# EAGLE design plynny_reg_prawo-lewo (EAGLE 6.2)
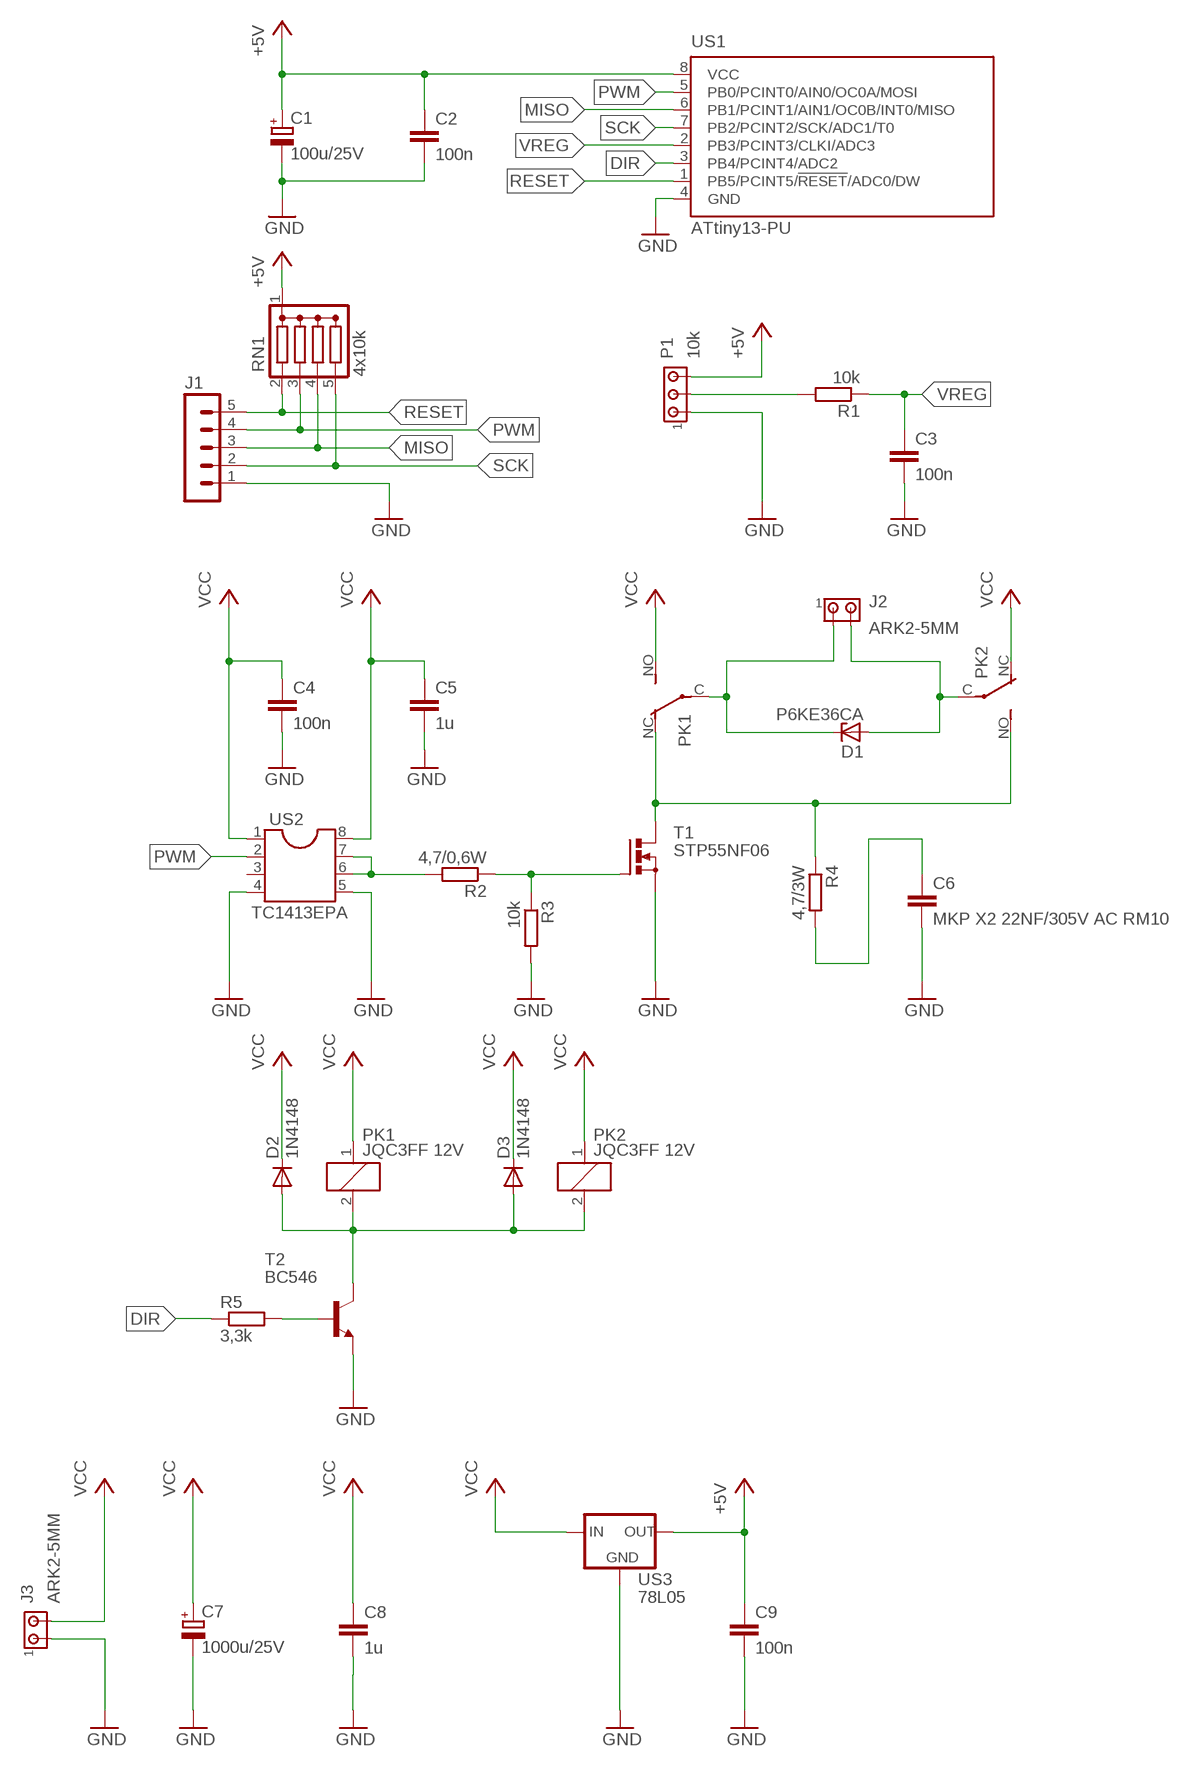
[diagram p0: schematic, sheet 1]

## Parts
C1  100u/25V  CPOL-EUE2.5-6  [E2,5-6]
C2  100n  C-EU050-025X075  [C050-025X075]
C3  100n  C-EU050-025X075  [C050-025X075]
C4  100n  C-EU050-025X075  [C050-025X075]
C5  1u  C-EU050-055X075  [C050-055X075]
C6  MKP X2 22NF/305V AC RM10  C-EU102-054X133  [C102-054X133]
C7  1000u/25V  CPOL-EUE5-10.5  [E5-10,5]
C8  1u  C-EU050-055X075  [C050-055X075]
C9  100n  C-EU050-025X075  [C050-025X075]
D1  P6KE36CA  ZENER-DIODEC1702-15  [C1702-15]
D2  1N4148  1N4148DO35-10  [DO35-10]
D3  1N4148  1N4148DO35-10  [DO35-10]
J1  MA05-1  [MA05-1]
J2  ARK2-5MM  [2PIN-5MM]
J3  ARK2-5MM  [2PIN-5MM]
P1  10k  ARK3-5MM  [3PIN-5MM]
PK1  JQC3FF 12V  PK_POJED-JQC-3FG  [PK_POJED_JQC-3FG]
PK2  JQC3FF 12V  PK_POJED-JQC-3FG  [PK_POJED_JQC-3FG]
R1  10k  R-EU_0207/7  [0207/7]
R2  4,7/0,6W  R-EU_0207/12  [0207/12]
R3  10k  R-EU_0207/7  [0207/7]
R4  4,7/3W  R-EU_R_18MM  [R_18MM]
R5  3,3k  R-EU_0207/7  [0207/7]
RN1  4x10k  DRAB_REZ_1X4  [RN-5]
T1  STP55NF06  BUZ11BV  [TO220BV]
T2  BC546  BC546A  [TO92-EBC]
US1  ATtiny13-PU  TINY13-20PU  [DIL08]
US2  TC1413EPA  DIL8  [DIL08]
US3  78L05  78LXX  [78LXX]

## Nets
+5V: C1.+ C2.1 C9.1 P1.P$3 RN1.1(C) US1.8(VCC) US3.OUT
DIR: R5.1 US1.3(PB4/PCINT4/ADC2)
GND: C1.- C2.2 C3.2 C4.2 C5.2 C6.2 C7.- C8.2 C9.2 J1.1 J3.P$1 P1.P$1 R3.2 T1.S T2.E US1.4(GND) US2.4 US2.5 US3.GND
MISO: J1.3 RN1.4 US1.6(PB1/PCINT1/AIN1/OC0B/INT0/MISO)
N$1: P1.P$2 R1.2
N$2: R2.2 US2.6 US2.7
N$3: PK1.NC PK2.NO R4.P$1 T1.D
N$4: C6.1 R4.P$2
N$5: R2.1 R3.1 T1.G
N$6: D1.C J2.P$1 PK1.C(COM)
N$7: D1.A J2.P$2 PK2.C(COM)
N$8: R5.2 T2.B
N$9: D2.A D3.A PK1.2 PK2.2 T2.C
PWM: J1.4 RN1.3 US1.5(PB0/PCINT0/AIN0/OC0A/MOSI) US2.2
RESET: J1.5 RN1.2 US1.1(PB5/PCINT5/!RESET!/ADC0/DW)
SCK: J1.2 RN1.5 US1.7(PB2/PCINT2/SCK/ADC1/T0)
VCC: C4.1 C5.1 C7.+ C8.1 D2.C D3.C J3.P$2 PK1.1 PK1.NO PK2.1 PK2.NC US2.1 US2.8 US3.IN
VREG: C3.1 R1.1 US1.2(PB3/PCINT3/CLKI/ADC3)
Unconnected: US2.3

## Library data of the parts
C1 C7 = rcl:CPOL-EU: POLARIZED CAPACITOR, European symbol
C2-C6 C8 C9 = rcl:C-EU: CAPACITOR, European symbol
D1 = diode:ZENER-DIODE: Z-Diode
D2 D3 = diode:1N4148: DIODE
J1 = con-lstb:MA05-1: PIN HEADER; OC_FARNELL: unknown; OC_NEWARK: unknown
J2 J3 = zlacza_futrzak:ARK2: ARK 2
P1 = zlacza_futrzak:ARK3: ARK 3 Raster 5mm i 3,5mm
PK1 PK2 = inne_futrzak:PK_POJED
R1-R5 = rcl:R-EU_: RESISTOR, European symbol
RN1 = inne_futrzak:DRAB_REZ_1X4
T1 = transistor-power:BUZ11: N-CHANNEL MOS FET
T2 = transistor-npn:BC546*: NPN Transistor
US1 = atmel:TINY13: 8-bit AVR Microcontroller with 1K Bytes In-System Programmable Flash Source: http://www.atmel.com/dyn/resources/prod_documents/2535S.pdf; MPN: ATTINY13-20PU; OC_FARNELL: 9171550; OC_NEWARK: 96K6521
US2 = ic-package:DIL8: Dual In Line / Socket
US3 = v-reg:78LXX: VOLTAGE REGULATOR

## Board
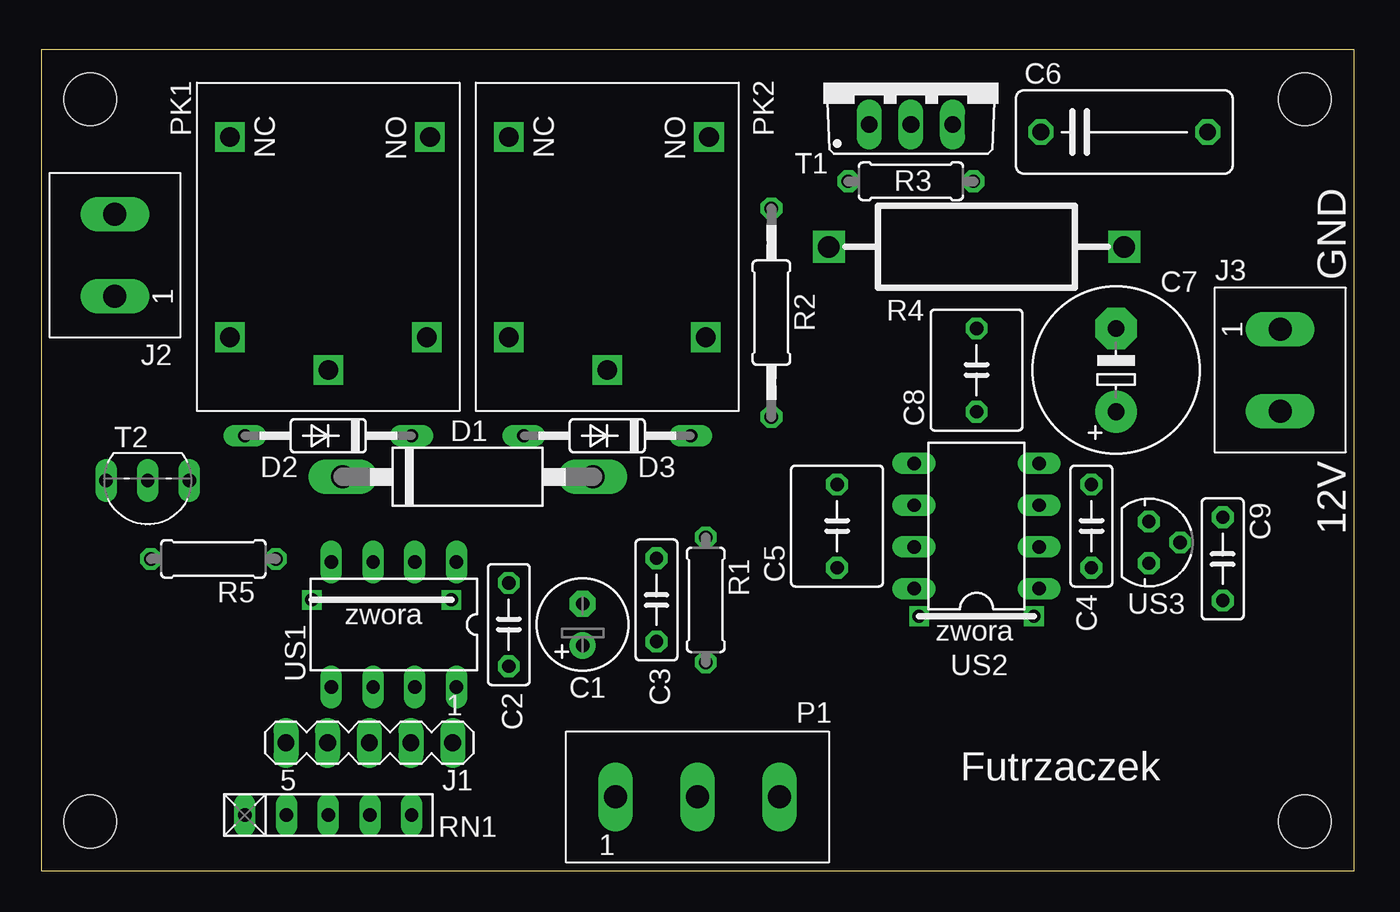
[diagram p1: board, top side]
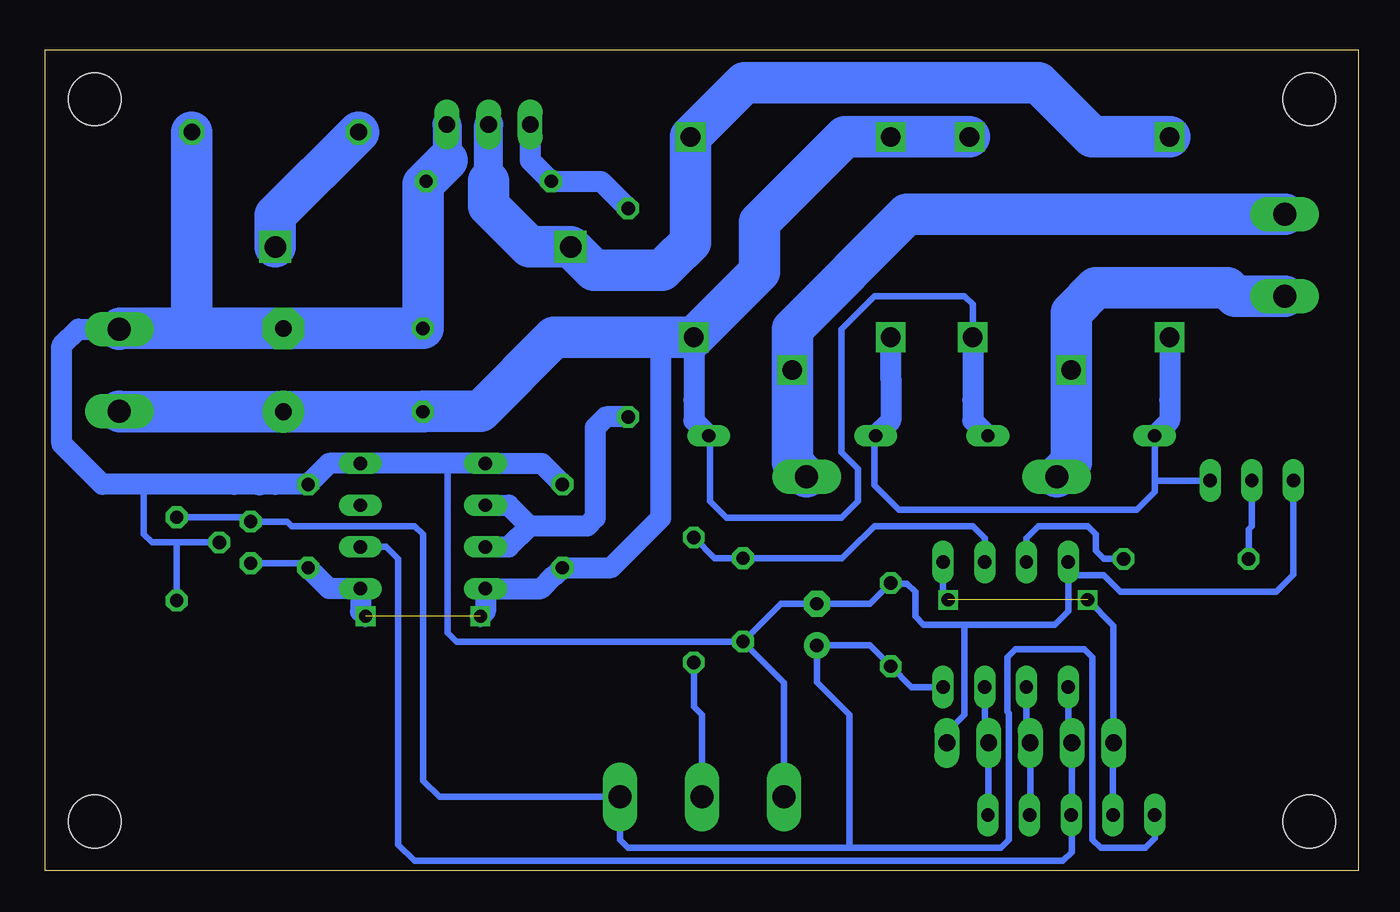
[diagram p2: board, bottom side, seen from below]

Size 80 x 50 mm. Coordinates in mm from the lower left corner, seen from the top.
Outline: 0,0 80,0 80,50 0,50 0,0
Copper layers (1*16): Top 0.035mm / dielectric 1.5mm / Bottom 0.035mm
Design rules: minimum track width 10mil, minimum drill 23mil, track to track 8mil, track to pad 8mil, pad to pad 8mil, via to via 8mil, smd to smd 8mil, copper to edge 10mil, drill to drill 8mil, minimum pad ring 10mil, minimum via ring 8mil, stop-mask expansion 4mil, vias tented up to drill 0mil, thermal gap 10mil
Holes 3.2 mm at 3,3 3,47 77,3 77,47

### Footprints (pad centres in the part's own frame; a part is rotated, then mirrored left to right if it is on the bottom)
E2,5-6 = drill 0.813 pad 1.6: + -1.27,0 | drill 0.813 pad 1.6 octagon: - 1.27,0
C050-025X075 = drill 0.813 octagon: 1 -2.54,0; 2 2.54,0
C050-055X075 = drill 0.813 octagon: 1 -2.54,0; 2 2.54,0
C102-054X133 = drill 1.016 octagon: 1 -5.08,0; 2 5.08,0
E5-10,5 = drill 1.016 pad 2.54: + -2.54,0 | drill 1.016 pad 2.54 octagon: - 2.54,0
C1702-15 = drill 1.397 long: A 7.62,0; C -7.62,0
DO35-10 = drill 0.813 long: A 5.08,0; C -5.08,0
MA05-1 = drill 1.016 long: 1 -5.08,0; 2 -2.54,0; 3 0,0; 4 2.54,0; 5 5.08,0
2PIN-5MM = drill 1.4 long: P$1 -2.5,0; P$2 2.5,0
3PIN-5MM = drill 1.4 long: P$1 -5,0; P$2 0,0; P$3 5,0
PK_POJED_JQC-3FG = drill 1.2 square: 1 5.5,6; 2 5.5,-6; C 7.5,0; NC -6.7,-6; NO -6.7,6.2
0207/7 = drill 0.813 octagon: 1 -3.81,0; 2 3.81,0
0207/12 = drill 0.813 octagon: 1 -6.35,0; 2 6.35,0
R_18MM = drill 1.3 square: P$1 -9,0; P$2 9,0
RN-5 = drill 0.813 long: 1 -5.08,0; 2 -2.54,0; 3 0,0; 4 2.54,0; 5 5.08,0
TO220BV = drill 1.016 long: D 0,-2.54; G -2.54,-2.54; S 2.54,-2.54
TO92-EBC = drill 0.813 long: B 0,-1.27; C -2.54,-1.27; E 2.54,-1.27
DIL08 = drill 0.813 long: 1 -3.81,-3.81; 2 -1.27,-3.81; 3 1.27,-3.81; 4 3.81,-3.81; 5 3.81,3.81; 6 1.27,3.81; 7 -1.27,3.81; 8 -3.81,3.81
78LXX = drill 0.813 octagon: GND 0,1.905; IN 1.27,0; OUT -1.27,0

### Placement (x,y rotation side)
C1  33,15 90 top
C2  28.5,15 90 top
C3  37.5,16.5 270 top
C4  64,21 90 top
C5  48.5,21 90 top
C6  66,45 0 top
C7  65.5,30.5 90 top
C8  57,30.5 90 top
C9  72,19 270 top
D1  26,24 0 top
D2  17.5,26.5 180 top
D3  34.5,26.5 180 top
J1  20,7.8 180 top
J2  4.5,37.5 90 top
J3  75.5,30.5 270 top
P1  40,4.5 0 top
PK1  17.5,38 270 top
PK2  34.5,38 270 top
R1  40.5,16.5 270 top
R2  44.5,34 270 top
R3  53,42 0 top
R4  57,38 0 top
R5  10.5,19 180 top
RN1  17.5,3.4 0 top
T1  53,48 0 top
T2  6.5,22.5 180 top
US1  21.5,15 180 top
US2  57,21 90 top
US3  67.5,20 270 top

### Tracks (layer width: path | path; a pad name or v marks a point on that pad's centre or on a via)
+5V
  Bottom 0.406: US1.8 27.23,11.19 C2.1 29.77,13.73 C1.+ 33,11.5 31,9.5 31,1.4 | RN1.1 12.42,1.98 13,1.4 15.7,1.4 16.2,1.9 16.2,13 16.7,13.5 20.3,13.5 20.9,13.5 21.4,13 21.4,9.7 21.3,9.6 21.3,1.9 21.8,1.4 31,1.4 | 31,1.4 44.5,1.4 45,1.9 P1.P$3 56,4.5 57,5.5 57,20.5 57.5,21 65,21 65.27,21.27 US3.OUT 67.77,21.54 C9.1
DIR
  Bottom 0.406: US1.3 20.23,20.27 19.5,21 16.5,21 16,20.5 16,19.5 15.5,19 R5.1
GND
  Bottom 0.406: US1.4 17.69,18 | 17.69,18 17.69,17.31 17.69,15.81 18.5,15 24,15 | 24,15 26.5,15 27,15.5 27,17 27.5,17.5 28.46,17.5 C2.2 29.77,16.27 C1.- 35.19,16.27 C3.2 | J1.1 25.08,8.42 24,9.5 24,15 | T2.E 3.96,18.04 5,17 14.5,17 15.5,18 17.69,18 | P1.P$1 35,11.46 C3.2 | C3.2 54.96,13.96 55.5,14.5 55.5,24.81 | US3.GND 72,20 | 72,20 73.5,20 74,20.5 74,23.54 | C9.2 72,20
  Bottom 1.27: C5.2 49.77,24.81 US2.5 55.5,24.81 US2.4 62.73,24.81 C4.2 66,23.54 67,23.54 | 67,23.54 68.5,23.54 74,23.54 76.54,23.54 79,26 79,32 78,33 J3.P$1 | 66.96,23.5 67,23.54
  Bottom 1.778: T1.S 55.54,43.27
  Bottom 2.54: 71.5,33.04 C7.- C8.2 57,41.81 R3.2 55.54,43.27 | 71.5,33.04 75.46,33.04 J3.P$1 | C6.2 71.08,33.46 71.5,33.04
MISO
  Bottom 0.406: US1.6 20.23,7.73 J1.3 20,3.04 RN1.4
N$1
  Bottom 0.406: P1.P$2 40,9.5 40.5,10 R1.2
N$2
  Bottom 1.27: R2.2 45.85,27.65 46.5,27 46.5,21.5 47,21 50.5,21 | US2.7 51.77,19.73 50.5,21 | US2.6 51.77,22.27 50.5,21
N$3
  Bottom 1.778: 53,42 T1.D
  Bottom 2.54: PK1.NC 16.2,44.7 18.5,47 19.5,48 37.4,48 PK2.NO 40.7,38.3 42,37 42.42,36.58 46.58,36.58 R4.P$1 50.5,38 53,40.5 53,42
N$4
  Bottom 2.54: R4.P$2 66,39.92 C6.1
N$5
  Bottom 1.27: T1.G 50.46,43.27 R3.1 46.15,42 R2.1
N$6
  Bottom 2.54: J2.P$1 7.5,35 8,35.5 16,35.5 17.5,34 PK1.C 17.5,24.88 D1.C
N$7
  Bottom 2.54: PK2.C 34.5,30 | 34.5,30 34.5,24.88 D1.A | J2.P$2 27.5,40 34.5,33 34.5,30
N$8
  Bottom 0.406: T2.B 6.5,21 6.69,20.81 R5.2
N$9
  Bottom 0.406: D2.A 12.42,25 | 12.42,25 12.42,23.08 13.5,22 28,22 29.5,23.5 29.5,26.42 D3.A | T2.C 12.42,23.77 12.42,25
  Bottom 1.27: PK1.2 11.5,28.69 11.5,27.42 D2.A | PK2.2 28.5,30 28.5,27.42 D3.A
PWM
  Bottom 0.406: US1.5 17.69,7.73 J1.4 17.46,3.04 | 17.46,3.04 RN1.3 17.46,3.04 | 17.46,3.04 17.46,1.14 18,0.6 57.5,0.6 58.5,1.6 58.5,19 59,19.5 59.23,19.73 US2.2
RESET  (via drill 0.8)  (1 unrouted)
  Bottom 0.406: RN1.2 14.96,7.46 J1.5 14.92,12.42 14.92,14.92 v16.5,16.5 | US1.1 25.31,16.81 v25,16.5
SCK
  Bottom 0.406: US1.7 22.77,7.73 J1.2 22.54,3.04 RN1.5
VCC  (via drill 0.8)  (1 unrouted)
  Bottom 0.406: PK1.1 23.5,34.5 24,35 29.5,35 31.5,33 31.5,25.5 30.5,24.5 30.5,22.5 31.5,21.5 38.5,21.5 39.5,22.5 39.5,26.42 D3.C | US3.IN 64.27,18.73 C4.1
  Bottom 1.27: 56.96,28 C8.1 | PK2.1 40.5,28.69 40.5,27.42 D3.C | PK1.1 23.5,28.69 23.5,27.42 D2.C | C4.1 62.73,17.19 US2.1 60.81,15.81 v60.5,15.5 | 42.5,32.5 42.5,21.5 45.54,18.46 C5.1 48.96,18 49,18 49.81,17.19 US2.8 53.19,15.81 v53.5,15.5
  Bottom 2.54: C8.1 C7.+ 75.46,27.96 J3.P$2 | 56.96,28 53.5,28 49,32.5 42.5,32.5 PK2.1 36.5,36.5 36.5,39.5 31.3,44.7 PK2.NC PK1.NO
VREG
  Bottom 0.406: US1.2 22.77,20.27 23.5,21 29.5,21 31,19.5 31.46,19.04 C3.1 39.23,19.04 R1.1

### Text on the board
tPlace: GND | 12V | zwora | zwora | Futrzaczek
